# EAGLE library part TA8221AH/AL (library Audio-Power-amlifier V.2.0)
30W BTLx2ch AUDIO POWER AMPLIEFIER
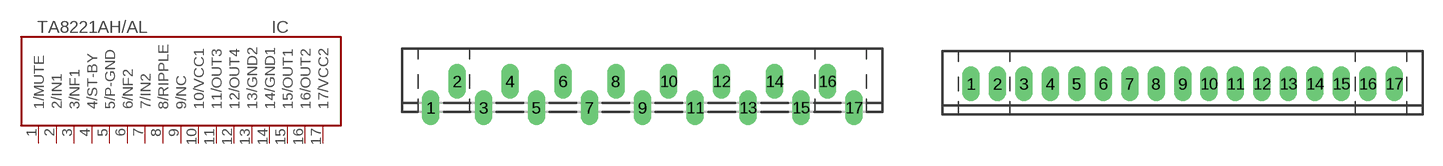
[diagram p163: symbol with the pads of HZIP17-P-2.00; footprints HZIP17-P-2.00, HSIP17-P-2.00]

Designator prefix IC

## TA8221AH/ALTA8221AH  [HZIP17-P-2.00]
1  1/MUTE  in
2  2/IN1  in
3  3/NF1  in
4  4/ST-BY  in
5  5/P-GND  pwr
6  6/NF2  in
7  7/IN2  in
8  8/RIPPLE
9  9/NC  nc
10  10/VCC1  pwr
11  11/OUT3  out
12  12/OUT4  out
13  13/GND2  pwr
14  14/GND1  pwr
15  15/OUT1  out
16  16/OUT2  out
17  17/VCC2  pwr

## TA8221AH/ALTA8221AL  [HSIP17-P-2.00]
Pads as for HZIP17-P-2.00

## Footprint HZIP17-P-2.00 (pad centres in mm)
HZIP17-P-2.00 Source: http://www.semicon.toshiba.co.jp/td/en/ASSP/Audio_ICs/en_20050517_TA8210ALQ_datasheet.pdf
drill 0.8 pad 1.2 long: 1 -16,-2; 2 -14,0; 3 -12,-2; 4 -10,0; 5 -8,-2; 6 -6,0; 7 -4,-2; 8 -2,0; 9 0,-2; 10 2,0; 11 4,-2; 12 6,0; 13 8,-2; 14 10,0; 15 12,-2; 16 14,0; 17 16,-2

## Footprint HSIP17-P-2.00 (pad centres in mm)
HSIP17-P-2.00 Source: http://www.semicon.toshiba.co.jp/td/en/ASSP/Audio_ICs/en_20050517_TA8210ALQ_datasheet.pdf
drill 0.8 pad 1.2 long: 1 -16,0; 2 -14,0; 3 -12,0; 4 -10,0; 5 -8,0; 6 -6,0; 7 -4,0; 8 -2,0; 9 0,0; 10 2,0; 11 4,0; 12 6,0; 13 8,0; 14 10,0; 15 12,0; 16 14,0; 17 16,0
